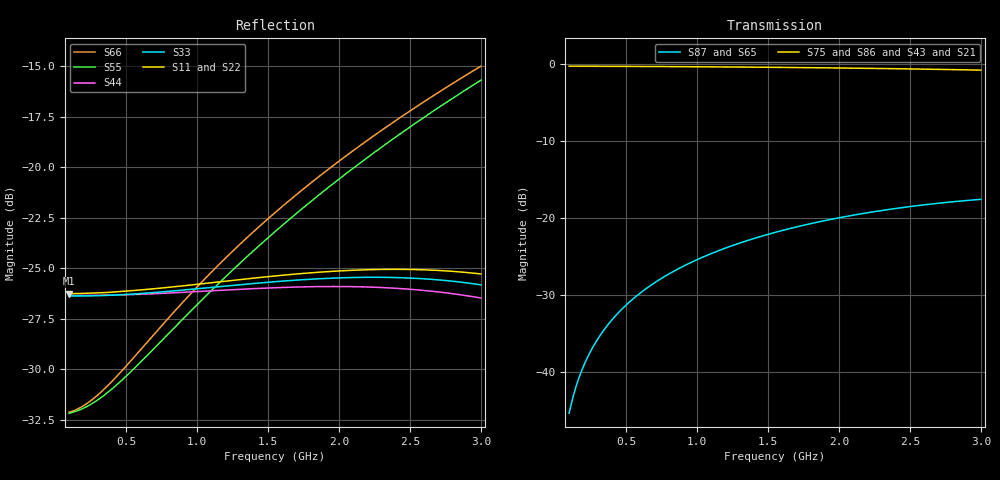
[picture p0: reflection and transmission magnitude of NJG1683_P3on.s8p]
! Created Wed May 22 11:49:10 2013
# hz S ma R 50
! 8 Port Network Data from SP2.SP block
! freq  magS11  angS11  magS12  angS12  magS13  angS13  magS14  angS14
!  magS15  angS15  magS16  angS16  magS17  angS17  magS18  angS18
!  magS21  angS21  magS22  angS22  magS23  angS23  magS24  angS24
!  magS25  angS25  magS26  angS26  magS27  angS27  magS28  angS28
!  magS31  angS31  magS32  angS32  magS33  angS33  magS34  angS34
!  magS35  angS35  magS36  angS36  magS37  angS37  magS38  angS38
!  magS41  angS41  magS42  angS42  magS43  angS43  magS44  angS44
!  magS45  angS45  magS46  angS46  magS47  angS47  magS48  angS48
!  magS51  angS51  magS52  angS52  magS53  angS53  magS54  angS54
!  magS55  angS55  magS56  angS56  magS57  angS57  magS58  angS58
!  magS61  angS61  magS62  angS62  magS63  angS63  magS64  angS64
!  magS65  angS65  magS66  angS66  magS67  angS67  magS68  angS68
!  magS71  angS71  magS72  angS72  magS73  angS73  magS74  angS74
!  magS75  angS75  magS76  angS76  magS77  angS77  magS78  angS78
!  magS81  angS81  magS82  angS82  magS83  angS83  magS84  angS84
!  magS85  angS85  magS86  angS86  magS87  angS87  magS88  angS88
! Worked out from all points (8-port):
!   291 points, 100 MHz to 3 GHz, reference 50 ohm
!   strongest paths, dB at 100 MHz, 820 MHz, 1.55 GHz, 2.28 GHz, 3 GHz:
!     S75: -0.3, -0.3, -0.4, -0.6, -0.8
!     S86: -0.3, -0.3, -0.4, -0.6, -0.8
!     S43: -0.5, -0.5, -0.5, -0.6, -0.6
!     S21: -0.5, -0.5, -0.5, -0.6, -0.6
!     S87: -45.3, -27.1, -21.8, -19.1, -17.6
!     S65: -45.2, -27.1, -21.9, -19.2, -17.7
!   lowest |S11| = -26.3 dB at 100 MHz (marker M1), VSWR 1.10, Z = 55.1 + j0.127 ohm
!   |S11| at or under -10 dB: start of sweep to end of sweep
